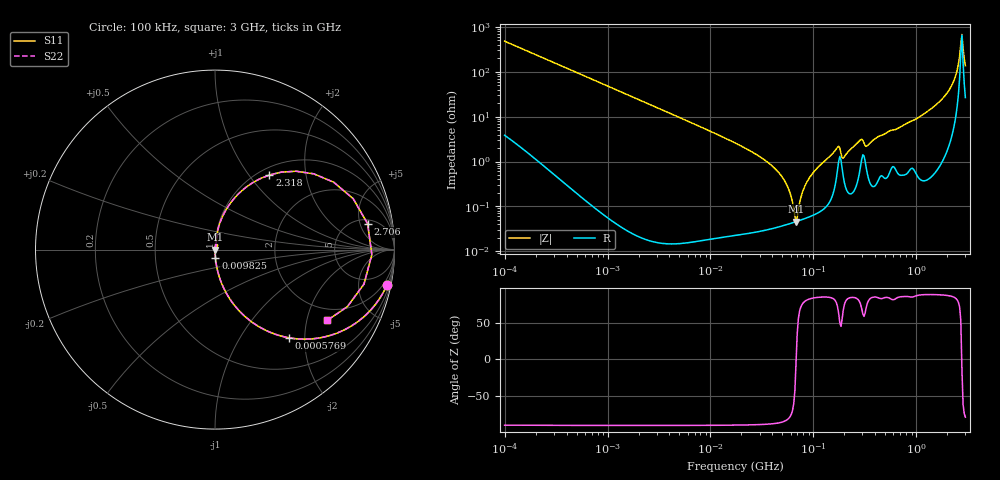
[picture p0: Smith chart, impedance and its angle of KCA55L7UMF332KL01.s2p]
!Murata Part Number: KCA55L7UMF332KL01
!These Parameters are Measured in Series Mode Connection
!Data Generated on Jan 08, 2026
!  o--ll--o
!Port1  Port2
!  o------o
!Operation Temp=25[degC], DC Bias Voltage=0[V]
!Freq. Start=100[kHz] Stop=3[GHz] 401[Steps]
# Hz S RI R 50
!Freq.(Hz) S11(Real) S11(Imag) S21(Real) S21(Imag) S12(Real) S12(Imag) S22(Real) S22(Imag)
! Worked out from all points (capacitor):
!   401 points, 100 kHz to 3 GHz, reference 50 ohm
!   read as one part in series: C = 3.31 nF near 105.3 kHz
!   lowest |Z| = 46 mohm at 67.89 MHz (marker M1)
!   series resonance near 68.09 MHz, so ESL is about 1.7 nH
!   S11 on the Smith chart (normalised r, x): 100 kHz: 1.08, -9.61; 576.9 kHz: 1.00, -1.67; 9.825 MHz: 1.00, -0.10; 2.318 GHz: 1.12, +1.26; 2.706 GHz: 5.98, +6.69; 3 GHz: 1.53, -2.67
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100000  0.957 -0.1989  0.043 0.1989  0.043 0.1989  0.957 -0.1989
234079  0.8081 -0.3918  0.1919 0.3918  0.1919 0.3918  0.8081 -0.3918
562235  0.4239 -0.4933  0.5761 0.4933  0.5761 0.4933  0.4239 -0.4933
576913  0.4114 -0.4912  0.5886 0.4912  0.5886 0.4912  0.4114 -0.4912
3161081  0.0228 -0.1487  0.9772 0.1487  0.9772 0.1487  0.0228 -0.1487
9824692  0.00248 -0.0479  0.9975 0.0479  0.9975 0.0479  0.00248 -0.0479
1.77727e7  0.000863 -0.0252  0.9991 0.0252  0.9991 0.0252  0.000863 -0.0252
4.611977e7  0.000381 -0.00564  0.9996 0.00564  0.9996 0.00564  0.000381 -0.00564
5.667996e7  0.000407 -0.00261  0.9996 0.00261  0.9996 0.00261  0.000407 -0.00261
6.788584e7  0.000458 -4.23e-05  0.9995 4.23e-05  0.9995 4.23e-05  0.000458 -4.23e-05
8.130716e7  0.000535 0.00254  0.9995 -0.00254  0.9995 -0.00254  0.000535 0.00254
9.738194e7  0.000649 0.00526  0.9994 -0.00526  0.9994 -0.00526  0.000649 0.00526
1.716802e8  0.0068 0.0195  0.9932 -0.0195  0.9932 -0.0195  0.0068 0.0195
2.003904e8  0.0035 0.0124  0.9965 -0.0124  0.9965 -0.0124  0.0035 0.0124
2.801453e8  0.0063 0.0279  0.9937 -0.0279  0.9937 -0.0279  0.0063 0.0279
3.355313e8  0.00562 0.0219  0.9944 -0.0219  0.9944 -0.0219  0.00562 0.0219
5.475153e8  0.00764 0.0468  0.9924 -0.0468  0.9924 -0.0468  0.00764 0.0468
1.701687e9  0.0539 0.2083  0.9461 -0.2083  0.9461 -0.2083  0.0539 0.2083
2.318426e9  0.303 0.4156  0.697 -0.4156  0.697 -0.4156  0.303 0.4156
2.504792e9  0.5497 0.4223  0.4503 -0.4223  0.4503 -0.4223  0.5497 0.4223
2.706139e9  0.8506 0.1432  0.1494 -0.1432  0.1494 -0.1432  0.8506 0.1432
3e9  0.6253 -0.3946  0.3747 0.3946  0.3747 0.3946  0.6253 -0.3946
